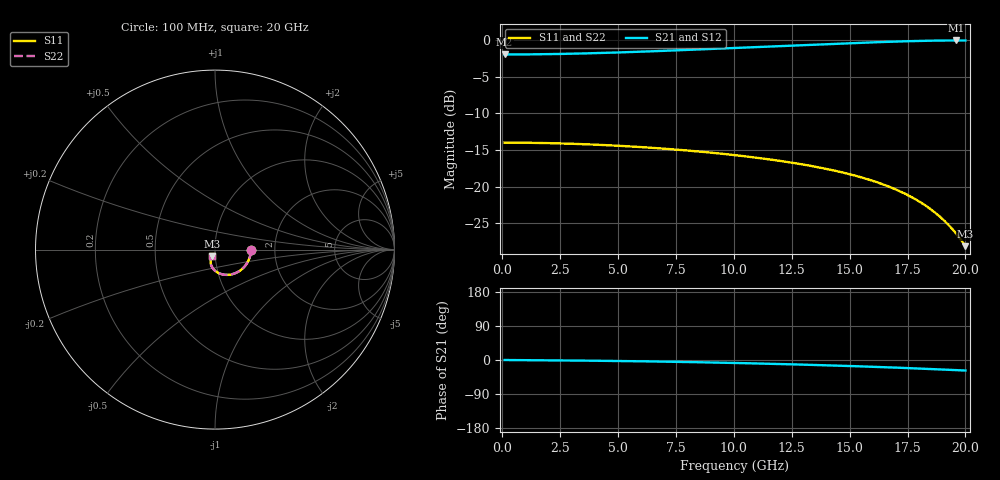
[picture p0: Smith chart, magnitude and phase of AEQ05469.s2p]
! Sonnet Data File
! From: emgraph Version : 16.52
! From Emgraph Data: AEQ05469_simulation_R5D
! Data File Written: 02/28/2018 09:15:53
!< HDATE 02/28/2018 09:13:10
!< MDATE 02/28/2018 09:13:10
# GHZ S MA R 50.00000
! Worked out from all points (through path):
!   200 points, 100 MHz to 20 GHz, reference 50 ohm
!   highest |S21| = -0.02 dB at 19.6 GHz (marker M1); lowest = -1.9 dB at 100 MHz (marker M2)
!   group delay of S21, straight-line fit = 3.77 ps
!   lowest |S11| = -28.1 dB at 20 GHz (marker M3), VSWR 1.08, Z = 48.3 - j3.47 ohm
!   |S11| at or under -10 dB: start of sweep to end of sweep
!   |S22| runs from -28.2 to -14.0 dB; largest |S21 - S12| = 0
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0.1  0.2 -0.6  0.8 -0.0  0.8 -0.0  0.2 -0.6
1.8  0.1987 -10.5  0.8036 -0.8  0.8036 -0.8  0.1986 -10.5
3.5  0.1952 -20.4  0.8133 -1.6  0.8133 -1.6  0.1951 -20.4
5.1  0.19 -29.7  0.827 -2.7  0.827 -2.7  0.1899 -29.6
6.8  0.1827 -39.4  0.8453 -4.1  0.8453 -4.1  0.1825 -39.3
8.5  0.1737 -49.1  0.8663 -5.9  0.8663 -5.9  0.1734 -49.0
10.1  0.1638 -58.3  0.8875 -7.9  0.8875 -7.9  0.1634 -58.2
11.9  0.1507 -68.7  0.9124 -10.5  0.9124 -10.5  0.1503 -68.7
13.4  0.138 -77.7  0.9334 -12.9  0.9334 -12.9  0.1375 -77.8
14.3  0.1292 -83.2  0.9459 -14.5  0.9459 -14.5  0.1287 -83.4
15.2  0.1194 -88.9  0.9581 -16.3  0.9581 -16.3  0.119 -89.3
16  0.1096 -94.2  0.9685 -17.9  0.9685 -17.9  0.1092 -94.6
16.7  0.1 -98.8  0.9771 -19.4  0.9771 -19.4  0.09971 -99.4
17.6  0.0861 -104.8  0.9867 -21.5  0.9867 -21.5  0.08589 -105.7
18  0.07927 -107.4  0.9903 -22.5  0.9903 -22.5  0.0791 -108.5
18.4  0.07201 -109.9  0.9933 -23.5  0.9933 -23.5  0.07189 -111.1
18.7  0.06628 -111.5  0.9951 -24.3  0.9951 -24.3  0.0662 -113.0
19  0.06033 -113.0  0.9965 -25.1  0.9965 -25.1  0.06028 -114.6
19.3  0.05416 -114.1  0.9973 -25.9  0.9973 -25.9  0.05413 -116.0
19.6  0.04782 -114.7  0.9977 -26.7  0.9977 -26.7  0.04779 -116.9
19.8  0.04352 -114.6  0.9976 -27.3  0.9976 -27.3  0.04347 -117.2
20  0.03921 -114.0  0.9972 -27.8  0.9972 -27.8  0.03912 -116.9
